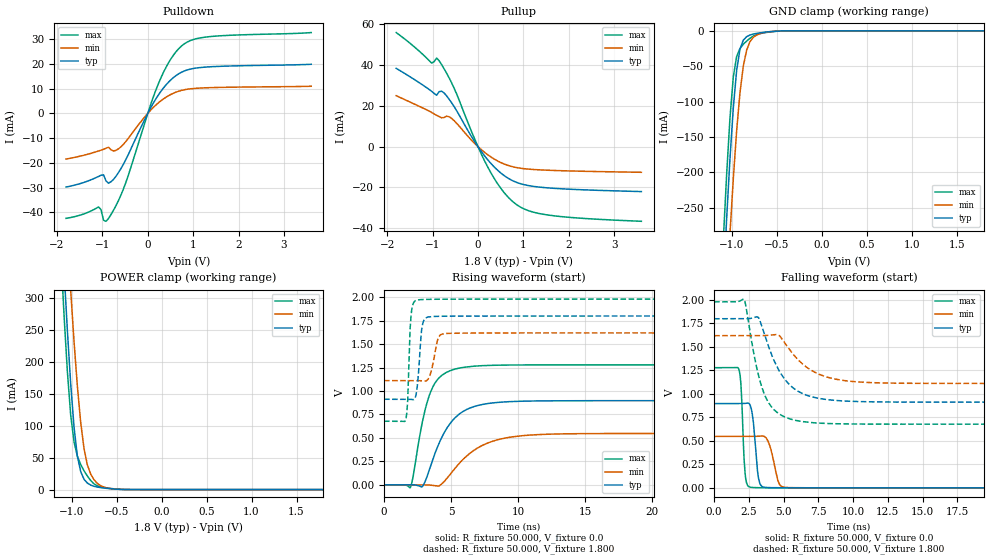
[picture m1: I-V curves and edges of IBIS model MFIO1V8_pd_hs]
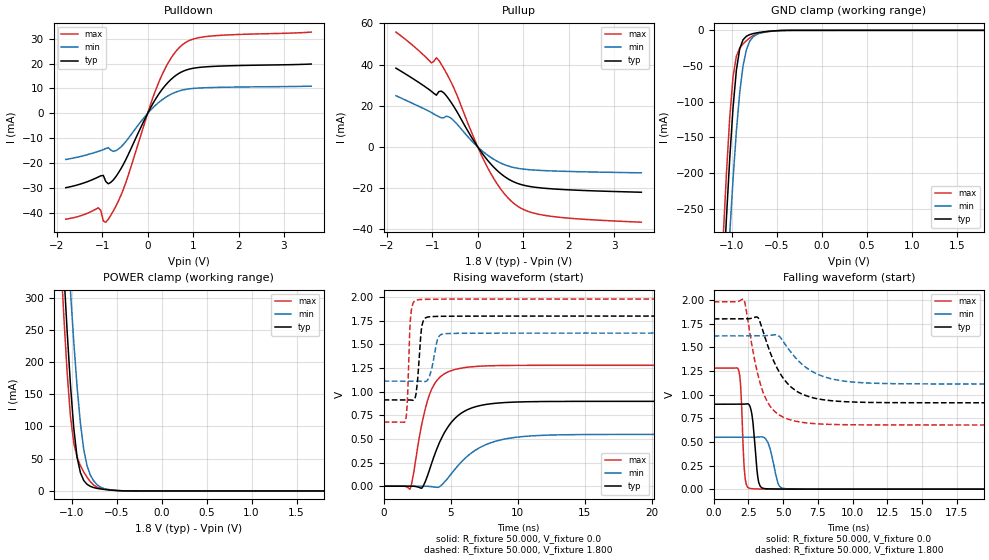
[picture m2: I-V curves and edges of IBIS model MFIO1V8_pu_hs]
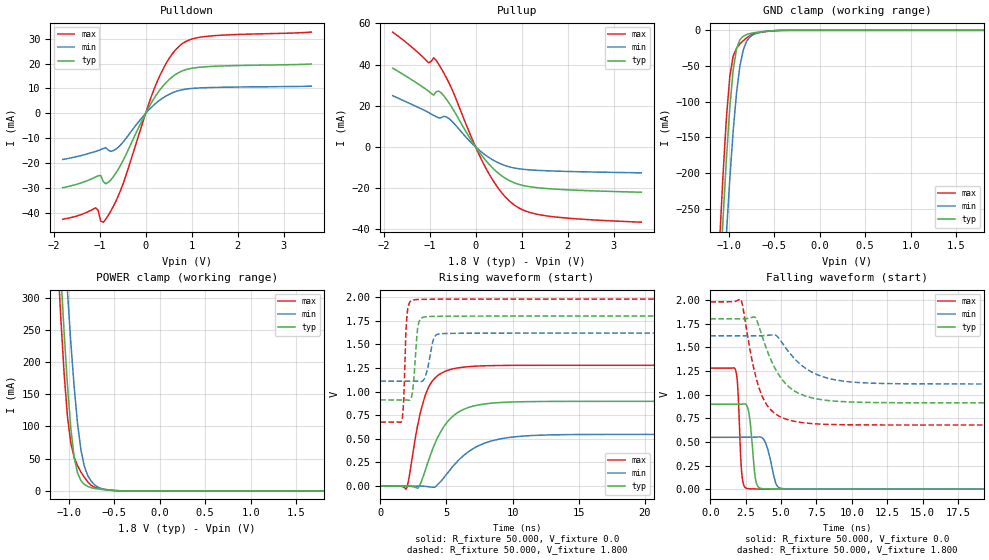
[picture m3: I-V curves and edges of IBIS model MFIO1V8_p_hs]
| IBIS file lpc55s6x_hlqfp100.ibs
[IBIS Ver]   5.0
[File name]   lpc55s6x_hlqfp100.ibs
[File Rev]   1.0
[Date]   January 29,2020
[Notes]   Rev History
|   1.0  initial release
[Disclaimer]   The model given below represents a 100-pin package.
[Copyright]   Copyright NXP 2020
|   Component lpc55s6x:hlqfp100
[Component] lpc55s6x
[Manufacturer] NXP
[Package]
|   typ   min   max
R_pkg   0.19438   0.14402   0.24011
L_pkg   4.719e-9   3.23e-9   5.804e-9
C_pkg   9.634e-13   4.793e-13   1.204e-12
[Pin]   Signal_name   model_name   R_pin   L_pin   C_pin
49   VBAT_DCDC   POWER   NA   NA   NA
50   VBAT_DCDC   POWER   NA   NA   NA
51   VBAT_PMU   POWER   NA   NA   NA
36   USB1_VBUS   POWER   NA   NA   NA
16   VDDA   POWER   NA   NA   NA
38   USB1_3V3   POWER   NA   NA   NA
96   USB0_3V3   POWER   NA   NA   NA
15   VDD   POWER   NA   NA   NA
25   VDD   POWER   NA   NA   NA
44   VDD   POWER   NA   NA   NA
63   VDD   POWER   NA   NA   NA
69   VDD   POWER   NA   NA   NA
75   VDD   POWER   NA   NA   NA
84   VDD   POWER   NA   NA   NA
95   VDD   POWER   NA   NA   NA
100   VDD   POWER   NA   NA   NA
39   VDD_PMU   POWER   NA   NA   NA
18   VREFN   NC   NA   NA   NA
17   VREFP   NC   NA   NA   NA
35   USB1_DM   NC   0.19961   3.9e-9   9.294e-13
34   USB1_DP   NC   0.20574   3.929e-9   9.444e-13
45   FB   NC   0.21411   3.71e-9   9.853e-13
48   LX   NC   0.14402   3.23e-9   1.143e-12
54   P0_0   gpio1v8   0.19671   5.046e-9   1.049e-12
7   P0_1   gpio1v8   0.18569   4.992e-9   9.758e-13
81   P0_2   gpio1v8   0.18955   4.93e-9   9.875e-13
83   P0_3   gpio1v8   0.20167   4.238e-9   9.373e-13
86   P0_4   gpio1v8   0.18453   4.604e-9   8.863e-13
88   P0_5   gpio1v8   0.17208   4.306e-9   4.861e-13
89   P0_6   gpio1v8   0.17688   4.76e-9   7.265e-13
6   P0_7   gpio1v8   0.18495   5.039e-9   9.877e-13
26   P0_8   gpio1v8   0.21082   5.764e-9   9.285e-13
55   P0_9   gpio1v8   0.18836   5.025e-9   1.013e-12
21   P0_10   gpio1v8   0.19767   4.742e-9   1.021e-12
13   P0_11   gpio1v8   0.16852   4.222e-9   4.793e-13
12   P0_12   gpio1v8   0.17445   4.737e-9   7.278e-13
71   P0_13   iicgpio1v8   0.20322   4.784e-9   1.026e-12
72   P0_14   iicgpio1v8   0.2062   5.002e-9   1.056e-12
22   P0_15   gpio1v8   0.20092   4.95e-9   1.063e-12
14   P0_16   gpio1v8   0.19182   3.934e-9   7.286e-13
8   P0_17   gpio1v8   0.18117   4.899e-9   9.571e-13
56   P0_18   gpio1v8   0.18284   4.955e-9   9.928e-13
90   P0_19   gpio1v8   0.17759   4.73e-9   8.974e-13
74   P0_20   gpio1v8   0.24011   4.357e-9   1.204e-12
76   P0_21   gpio1v8   0.21092   5.779e-9   9.242e-13
20   P0_22   gpio1v8   0.20457   4.183e-9   9.919e-13
78   P0_23   gpio1v8   0.19658   5.322e-9   1.084e-12
70   P0_24   gpio1v8   0.21211   4.242e-9   9.876e-13
79   P0_25   gpio1v8   0.19312   5.22e-9   1.048e-12
27   P0_26   gpio1v8   0.197   5.359e-9   1.171e-12
60   P0_27   gpio1v8   0.17389   4.719e-9   9.122e-13
66   P0_28   gpio1v8   0.18341   4.705e-9   9.109e-13
92   P0_9   gpio1v8   0.18226   4.694e-9   9.27e-13
23   P0_30   gpio1v8   0.21051   4.951e-9   1.105e-12
94   P0_31   gpio1v8   0.20907   4.051e-9   9.845e-13
11   P1_0   gpio1v8   0.17643   4.76e-9   9.003e-13
59   P1_1   gpio1v8   0.17508   4.772e-9   9.158e-13
61   P1_2   gpio1v8   0.17391   4.681e-9   9e-13
62   P1_3   gpio1v8   0.17584   4.65e-9   7.307e-13
1   P1_4   gpio1v8   0.21145   5.804e-9   9.228e-13
31   P1_5   gpio1v8   0.1979   4.791e-9   1.002e-12
5   P1_6   gpio1v8   0.19021   5.17e-9   1.023e-12
9   P1_7   gpio1v8   0.17814   4.834e-9   9.098e-13
10   P1_8   gpio1v8   0.1792   4.817e-9   9.052e-13
24   P1_9   gpio1v8   0.22787   4.483e-9   1.184e-12
40   P1_10   gpio1v8   0.19298   4.016e-9   8.906e-13
93   P1_11   gpio1v8   0.19014   4.583e-9   9.519e-13
67   P1_12   gpio1v8   0.19991   4.733e-9   9.253e-13
2   P1_13   gpio1v8   0.19954   5.432e-9   1.175e-12
57   P1_14   gpio1v8   0.17887   4.872e-9   9.721e-13
82   P1_15   gpio1v8   0.1908   4.68e-9   9.803e-13
43   P1_16   gpio1v8   0.20312   4.087e-9   9.402e-13
87   P1_17   gpio1v8   0.18016   4.71e-9   7.274e-13
64   P1_18   gpio1v8   0.17645   4.681e-9   7.229e-13
58   P1_19   gpio1v8   0.1767   4.814e-9   9.428e-13
4   P1_20   gpio1v8   0.19631   5.293e-9   1.056e-12
30   P1_21   gpio1v8   0.19856   5.07e-9   1.02e-12
41   P1_22   gpio1v8   0.18488   4.442e-9   9.08e-13
42   P1_23   gpio1v8   0.18716   4.441e-9   9.092e-13
3   P1_24   gpio1v8   0.20078   5.394e-9   1.079e-12
77   P1_25   gpio1v8   0.19946   5.414e-9   1.191e-12
68   P1_26   gpio1v8   0.20751   4.306e-9   9.447e-13
85   P1_27   gpio1v8   0.19867   4.289e-9   8.839e-13
73   P1_28   gpio1v8   0.21386   4.888e-9   1.092e-12
65   P1_29   gpio1v8   0.17885   4.696e-9   9.052e-13
80   P1_30   gpio1v8   0.18891   5.065e-9   1.012e-12
91   P1_31   gpio1v8   0.17881   4.709e-9   9.248e-13
32   RESETN   gpio1v8   0.2115   4.197e-9   9.778e-13
97   USB0_DP   NC   0.22563   4.185e-9   1.051e-12
98   USB0_DM   NC   0.23166   4.181e-9   1.087e-12
53   XTAL32K_N   NC   0.20814   4.918e-9   1.089e-12
52   XTAL32K_P   NC   0.23349   4.374e-9   1.189e-12
28   XTAL32M_N   NC   0.20639   5.416e-9   1.083e-12
29   XTAL32M_P   NC   0.20019   5.253e-9   1.052e-12
101   VSS   GND   NA   NA   NA
19   VSSA   GND   NA   NA   NA
33   USB1_VSS   GND   NA   NA   NA
37   USB1_VSS   GND   NA   NA   NA
47   VSS_DCDC   GND   NA   NA   NA
46   VSS_DCDC   GND   NA   NA   NA
99   USB0_VSS   GND   NA   NA   NA
|   Model Selector
[Model Selector] gpio1v8
MFIO1V8_pd_hs  EPUN=1 EPD=1 EHS=1
MFIO1V8_pd_ls  EPUN=1 EPD=1 EHS=0
MFIO1V8_pu_hs  EPUN=0 EPD=0 EHS=1
MFIO1V8_pu_ls  EPUN=0 EPD=0 EHS=0
MFIO1V8_p_hs  EPUN=1 EPD=0 EHS=1
MFIO1V8_p_ls  EPUN=1 EPD=0 EHS=0
MFIO1V8_r_hs  EPUN=0 EPD=1 EHS=1
MFIO1V8_r_ls  EPUN=0 EPD=1 EHS=0
[Model Selector] iicgpio1v8
IIC1V8_pd_hs  EGP=1 EPUN=1 EPD=1 EHS=1
IIC1V8_pd_ls  EGP=1 EPUN=1 EPD=1 EHS=0
IIC1V8_p_hs  EGP=1 EPUN=1 EPD=0 EHS=1
IIC1V8_p_ls  EGP=1 EPUN=1 EPD=0 EHS=0
IIC1V8_pu_hs  EGP=1 EPUN=0 EPD=0 EHS=1
IIC1V8_pu_ls  EGP=1 EPUN=0 EPD=0 EHS=0
IIC1V8_r_hs  EGP=1 EPUN=0 EPD=1 EHS=1
IIC1V8_r_ls  EGP=1 EPUN=0 EPD=1 EHS=0
IIC1V8_pd_iic_hs  EGP=0 ECS=0 EPUN=1 EPD=1
IIC1V8_p_iic_hs  EGP=0 ECS=0 EPUN=1 EPD=0
IIC1V8_pu_iic_hs  EGP=0 ECS=0 EPUN=0 EPD=0
IIC1V8_r_iic_hs  EGP=0 ECS=0 EPUN=0 EPD=1
IIC1V8_pd_iic_pu_hs  EGP=0 ECS=1 EPUN=1 EPD=1  SSEL=1
IIC1V8_p_iic_pu_hs  EGP=0 ECS=1 EPUN=1 EPD=0  SSEL=1
IIC1V8_pu_iic_pu_hs  EGP=0 ECS=1 EPUN=0 EPD=0  SSEL=1
IIC1V8_r_iic_pu_hs  EGP=0 ECS=1 EPUN=0 EPD=1  SSEL=1
| Models and submodels in the file (24): MFIO1V8_pd_hs (I/O), MFIO1V8_pd_ls (I/O), MFIO1V8_pu_hs (I/O), MFIO1V8_pu_ls (I/O), MFIO1V8_p_hs (I/O), MFIO1V8_p_ls (I/O), MFIO1V8_r_hs (I/O), MFIO1V8_r_ls (I/O), IIC1V8_pd_hs (I/O), IIC1V8_pd_ls (I/O), IIC1V8_p_hs (I/O), IIC1V8_p_ls (I/O), IIC1V8_pu_hs (I/O), IIC1V8_pu_ls (I/O), IIC1V8_r_hs (I/O), IIC1V8_r_ls (I/O), IIC1V8_pd_iic_hs (I/O_open_drain), IIC1V8_p_iic_hs (I/O_open_drain), IIC1V8_pu_iic_hs (I/O_open_drain), IIC1V8_r_iic_hs (I/O_open_drain), IIC1V8_pd_iic_pu_hs (I/O_open_drain), IIC1V8_p_iic_pu_hs (I/O_open_drain), IIC1V8_pu_iic_pu_hs (I/O_open_drain), IIC1V8_r_iic_pu_hs (I/O_open_drain)
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|   Model MFIO1V8_pd_hs
[Model] MFIO1V8_pd_hs
Model_type I/O
Polarity   Non-Inverting
Enable   Active-Low
Vinl =  0.540V
Vinh =  1.260V
Vmeas =  0.900V
Cref =  0.0F
Rref =  100.000
Vref =  0.0V
C_comp   2.019pF   1.989pF   2.068pF
C_comp_pullup   1.198pF   1.161pF   1.251pF
C_comp_pulldown   0.670pF   0.661pF   0.684pF
[Model Spec]
Vinh   1.260V   1.134V   1.386V
Vinl   0.540V   0.486V   0.594V
Vmeas   0.900V   0.810V   0.990V
Vref   0.0V   0.0V   0.0V
Cref   0.0F   0.0F   0.0F
Rref   100.000   100.000   100.000
[Temperature Range]   25.000   0.125k   -40.000
[Voltage Range]   1.800V   1.620V   1.980V
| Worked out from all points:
|   slope of the pulldown table from 0 to 0.27 V, typ, clamps not added: 32.2 ohm
|   slope of the pullup table from 0 to 0.27 V, typ, clamps not added: 34.3 ohm
|   GND clamp passes 1 mA (typ) near -0.56 V on its own axis
|   POWER clamp passes 1 mA (typ) near -0.54 V on its own axis
|   rising waveform, R_fixture 50.000, V_fixture 0.0: 20-80 % time 1.89ns typ, 2.69ns min, 1.21ns max; typ from 0 V to 0.897 V
|   rising waveform, R_fixture 50.000, V_fixture 1.800: 20-80 % time 276ps typ, 422ps min, 194ps max; typ from 0.912 V to 1.8 V
|   falling waveform, R_fixture 50.000, V_fixture 0.0: 20-80 % time 315ps typ, 502ps min, 217ps max; typ from 0.897 V to 0 V
|   falling waveform, R_fixture 50.000, V_fixture 1.800: 20-80 % time 1.84ns typ, 2.3ns min, 1.28ns max; typ from 1.8 V to 0.912 V
[Pulldown]
|Voltage   I(typ)   I(min)   I(max)
-1.8V     -29.75mA   -18.45mA   -42.39mA
-1.085V   -25.48mA   -15.2mA    -37.79mA
-1.03V    -24.99mA   -14.87mA   -38.88mA
-975mV    -24.83mA   -14.51mA   -43.15mA
-865mV    -28.18mA   -13.68mA   -42.43mA
-700mV    -25.38mA   -14.92mA   -37.23mA
-480mV    -18.54mA   -11.29mA   -27.73mA
235mV     7.474mA    4.265mA    12.03mA
510mV     13.55mA    7.648mA    22.01mA
785mV     16.96mA    9.446mA    27.8mA
1.39V     18.81mA    10.38mA    31.01mA
3.6V      19.8mA     10.93mA    32.61mA
[Pullup]
|Voltage   I(typ)   I(min)   I(max)
-1.8V     38.29mA    24.9mA     55.82mA
-1.02V    27.05mA    16.71mA    40.87mA
-910mV    25.14mA    15.31mA    43.32mA
-855mV    26.89mA    14.69mA    42.04mA
-745mV    26.24mA    14.22mA    38.06mA
-580mV    21.45mA    13.82mA    31.22mA
190mV     -5.761mA   -3.564mA   -8.914mA
520mV     -13.24mA   -7.997mA   -20.92mA
795mV     -17.02mA   -10.03mA   -27.47mA
1.07V     -18.92mA   -10.95mA   -31.04mA
1.51V     -20.18mA   -11.56mA   -33.41mA
3.6V      -22.04mA   -12.6mA    -36.6mA
[GND_clamp]
|Voltage   I(typ)   I(min)   I(max)
-1.8V     -2.463A    -2.494A    -2.446A
-1.097V   -357.7mA   -460.7mA   -294.8mA
-1.06V    -264.9mA   -370.9mA   -202.5mA
-1.023V   -180.4mA   -286.3mA   -122.9mA
-986mV    -108.7mA   -208.9mA   -65.05mA
-949mV    -56.06mA   -141.4mA   -36.24mA
-912mV    -25.87mA   -87.65mA   -25.01mA
-875mV    -13.21mA   -49.99mA   -19.06mA
-838mV    -8.315mA   -27.44mA   -14.52mA
-764mV    -4.558mA   -9.219mA   -7.395mA
-542mV    -813.9uA   -810.7uA   -1.086mA
1.8V      0A         0A         0A
[POWER_clamp]
|Voltage   I(typ)   I(min)   I(max)
-1.8V     2.577A     2.626A     2.553A
-1.123V   442.8mA    582.7mA    371.8mA
-1.086V   342mA      487.8mA    272.2mA
-1.049V   248.2mA    396.7mA    184.1mA
-1.012V   164.7mA    310.5mA    115.9mA
-975mV    97.4mA     231.2mA    74.47mA
-938mV    52.21mA    161.5mA    52.2mA
-864mV    16.15mA    64.06mA    29.43mA
-790mV    7.073mA    24.26mA    14.23mA
-679mV    3.152mA    6.087mA    4.407mA
-494mV    590.1uA    655.5uA    758.5uA
1.8V      0A         0A         0A
[Ramp]
| variable   typ   min   max
dV/dt_r   0.538/1.890n   0.328/2.680n   0.767/1.209n
dV/dt_f   0.532/1.835n   0.305/2.291n   0.781/1.275n
R_load = 50.000
[Rising Waveform]
R_fixture= 50.000
V_fixture= 0.0
V_fixture_min= 0.0
V_fixture_max= 0.0
|time   V(typ)   V(min)   V(max)
0s        6.721nV    117.6nV    4.416nV
1.96ns    159.2uV    -62.09nV   -31.69mV
2.85ns    -21.07mV   134.7uV    661mV
3.65ns    271.3mV    -6.708mV   1.047V
4.15ns    457.1mV    -8.65mV    1.146V
4.97ns    661.3mV    117.8mV    1.218V
6.65ns    830.9mV    361.7mV    1.264V
9.15ns    884.8mV    501.2mV    1.276V
13.74ns   896.1mV    543.8mV    1.278V
100ns     896.7mV    547.4mV    1.278V
[Rising Waveform]
R_fixture= 50.000
V_fixture= 1.800
V_fixture_min= 1.620
V_fixture_max= 1.980
|time   V(typ)   V(min)   V(max)
0s        911.9mV    1.111V     677.7mV
1.63ns    911.9mV    1.111V     697.7mV
1.77ns    912.1mV    1.111V     900.3mV
2.05ns    909.6mV    1.111V     1.849V
2.42ns    983.6mV    1.111V     1.967V
2.68ns    1.419V     1.11V      1.973V
3.06ns    1.772V     1.105V     1.976V
4.08ns    1.796V     1.575V     1.978V
4.84ns    1.798V     1.614V     1.979V
100ns     1.799V     1.619V     1.979V
[Falling Waveform]
R_fixture= 50.000
V_fixture= 0.0
V_fixture_min= 0.0
V_fixture_max= 0.0
|time   V(typ)   V(min)   V(max)
0s        896.7mV    547.4mV    1.278V
1.79ns    896.7mV    547.4mV    1.258V
1.93ns    896.6mV    547.4mV    1.106V
2.24ns    898.4mV    547.4mV    142.2mV
2.74ns    796.7mV    547.3mV    4.509mV
3.2ns     100.7mV    550.1mV    1.658mV
3.81ns    3.552mV    517mV      778.9uV
4.65ns    1.171mV    54.78mV    345.8uV
5.34ns    645.9uV    3.088mV    186.5uV
100ns     14.3nV     131.2nV    8.877nV
[Falling Waveform]
R_fixture= 50.000
V_fixture= 1.800
V_fixture_min= 1.620
V_fixture_max= 1.980
|time   V(typ)   V(min)   V(max)
0s        1.799V     1.619V     1.979V
2.17ns    1.799V     1.619V     2.003V
3.18ns    1.813V     1.619V     1.21V
3.88ns    1.522V     1.623V     915.7mV
4.62ns    1.262V     1.626V     793.3mV
5.16ns    1.14V      1.527V     750mV
6.98ns    971mV      1.252V     694.9mV
9.25ns    925.2mV    1.144V     680.9mV
13.25ns   913mV      1.113V     677.9mV
100ns     911.9mV    1.111V     677.7mV
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|   Model MFIO1V8_pu_hs
[Model] MFIO1V8_pu_hs
Model_type I/O
Polarity   Non-Inverting
Enable   Active-Low
Vinl =  0.540V
Vinh =  1.260V
Vmeas =  0.900V
Cref =  0.0F
Rref =  100.000
Vref =  0.0V
C_comp   2.019pF   1.989pF   2.068pF
C_comp_pullup   1.197pF   1.159pF   1.249pF
C_comp_pulldown   0.671pF   0.662pF   0.686pF
[Model Spec]
Vinh   1.260V   1.134V   1.386V
Vinl   0.540V   0.486V   0.594V
Vmeas   0.900V   0.810V   0.990V
Vref   0.0V   0.0V   0.0V
Cref   0.0F   0.0F   0.0F
Rref   100.000   100.000   100.000
[Temperature Range]   25.000   0.125k   -40.000
[Voltage Range]   1.800V   1.620V   1.980V
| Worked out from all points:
|   slope of the pulldown table from 0 to 0.27 V, typ, clamps not added: 32.2 ohm
|   slope of the pullup table from 0 to 0.27 V, typ, clamps not added: 34.3 ohm
|   GND clamp passes 1 mA (typ) near -0.56 V on its own axis
|   POWER clamp passes 1 mA (typ) near -0.54 V on its own axis
|   rising waveform, R_fixture 50.000, V_fixture 0.0: 20-80 % time 1.89ns typ, 2.68ns min, 1.21ns max; typ from 0.001 V to 0.898 V
|   rising waveform, R_fixture 50.000, V_fixture 1.800: 20-80 % time 275ps typ, 425ps min, 197ps max; typ from 0.913 V to 1.8 V
|   falling waveform, R_fixture 50.000, V_fixture 0.0: 20-80 % time 314ps typ, 505ps min, 216ps max; typ from 0.898 V to 0.001 V
|   falling waveform, R_fixture 50.000, V_fixture 1.800: 20-80 % time 1.84ns typ, 2.3ns min, 1.27ns max; typ from 1.8 V to 0.913 V
[Pulldown]
|Voltage   I(typ)   I(min)   I(max)
-1.8V     -29.75mA   -18.45mA   -42.39mA
-1.085V   -25.48mA   -15.2mA    -37.79mA
-1.03V    -24.99mA   -14.87mA   -38.88mA
-975mV    -24.83mA   -14.51mA   -43.15mA
-865mV    -28.18mA   -13.68mA   -42.43mA
-700mV    -25.38mA   -14.92mA   -37.23mA
-480mV    -18.54mA   -11.29mA   -27.73mA
235mV     7.474mA    4.265mA    12.03mA
510mV     13.55mA    7.648mA    22.01mA
785mV     16.96mA    9.446mA    27.8mA
1.39V     18.81mA    10.38mA    31.01mA
3.6V      19.8mA     10.93mA    32.61mA
[Pullup]
|Voltage   I(typ)   I(min)   I(max)
-1.8V     38.29mA    24.9mA     55.82mA
-1.02V    27.05mA    16.71mA    40.87mA
-910mV    25.14mA    15.31mA    43.32mA
-855mV    26.89mA    14.69mA    42.04mA
-745mV    26.24mA    14.22mA    38.06mA
-580mV    21.45mA    13.82mA    31.22mA
190mV     -5.761mA   -3.564mA   -8.914mA
520mV     -13.24mA   -7.997mA   -20.92mA
795mV     -17.02mA   -10.03mA   -27.47mA
1.07V     -18.92mA   -10.95mA   -31.04mA
1.51V     -20.18mA   -11.56mA   -33.41mA
3.6V      -22.04mA   -12.6mA    -36.6mA
[GND_clamp]
|Voltage   I(typ)   I(min)   I(max)
-1.8V     -2.463A    -2.494A    -2.446A
-1.097V   -357.7mA   -460.7mA   -294.9mA
-1.06V    -264.9mA   -371mA     -202.6mA
-1.023V   -180.4mA   -286.4mA   -122.9mA
-986mV    -108.7mA   -208.9mA   -65.09mA
-949mV    -56.09mA   -141.5mA   -36.28mA
-912mV    -25.91mA   -87.68mA   -25.06mA
-875mV    -13.24mA   -50.02mA   -19.11mA
-838mV    -8.35mA    -27.47mA   -14.57mA
-764mV    -4.593mA   -9.247mA   -7.441mA
-542mV    -849.5uA   -838.5uA   -1.132mA
1.8V      0A         0A         0A
[POWER_clamp]
|Voltage   I(typ)   I(min)   I(max)
-1.8V     2.577A     2.626A     2.553A
-1.123V   442.8mA    582.7mA    371.7mA
-1.086V   342mA      487.8mA    272.2mA
-1.049V   248.2mA    396.7mA    184.1mA
-1.012V   164.7mA    310.5mA    115.9mA
-975mV    97.36mA    231.1mA    74.42mA
-938mV    52.18mA    161.5mA    52.15mA
-864mV    16.11mA    64.03mA    29.39mA
-790mV    7.037mA    24.23mA    14.18mA
-679mV    3.116mA    6.059mA    4.361mA
-494mV    554.4uA    627.7uA    712.3uA
1.8V      0A         0A         0A
[Ramp]
| variable   typ   min   max
dV/dt_r   0.538/1.890n   0.329/2.680n   0.767/1.209n
dV/dt_f   0.532/1.835n   0.305/2.290n   0.781/1.276n
R_load = 50.000
[Rising Waveform]
R_fixture= 50.000
V_fixture= 0.0
V_fixture_min= 0.0
V_fixture_max= 0.0
|time   V(typ)   V(min)   V(max)
0s        630.6uV    679.1uV    587.5uV
1.96ns    789.2uV    678.8uV    -30.05mV
2.85ns    -19.7mV    812.3uV    661.1mV
3.62ns    261mV      -5.421mV   1.04V
4.13ns    453.5mV    -9.012mV   1.145V
4.91ns    652mV      107.5mV    1.216V
6.6ns     829.9mV    358mV      1.264V
9.06ns    885.4mV    500.2mV    1.277V
13.76ns   897.4mV    545.1mV    1.28V
100ns     898mV      548.7mV    1.28V
[Rising Waveform]
R_fixture= 50.000
V_fixture= 1.800
V_fixture_min= 1.620
V_fixture_max= 1.980
|time   V(typ)   V(min)   V(max)
0s        913.3mV    1.112V     678.9mV
1.63ns    913.3mV    1.112V     698.4mV
1.75ns    913.5mV    1.112V     853.9mV
2.02ns    911.7mV    1.112V     1.814V
2.4ns     967.4mV    1.112V     1.968V
2.67ns    1.397V     1.111V     1.974V
3.06ns    1.773V     1.107V     1.977V
4.07ns    1.797V     1.574V     1.979V
4.83ns    1.798V     1.615V     1.98V
100ns     1.8V       1.62V      1.98V
[Falling Waveform]
R_fixture= 50.000
V_fixture= 0.0
V_fixture_min= 0.0
V_fixture_max= 0.0
|time   V(typ)   V(min)   V(max)
0s        898mV      548.7mV    1.28V
1.79ns    898mV      548.7mV    1.259V
1.93ns    897.9mV    548.6mV    1.108V
2.24ns    899.8mV    548.7mV    143.9mV
2.76ns    775.9mV    548.5mV    5.275mV
3.23ns    78.56mV    551.7mV    2.369mV
3.84ns    4.35mV     511.3mV    1.439mV
4.67ns    1.941mV    48.66mV    967uV
5.32ns    1.374mV    4.206mV    798.7uV
100ns     630.7uV    679.1uV    587.5uV
[Falling Waveform]
R_fixture= 50.000
V_fixture= 1.800
V_fixture_min= 1.620
V_fixture_max= 1.980
|time   V(typ)   V(min)   V(max)
0s        1.8V       1.62V      1.98V
2.16ns    1.8V       1.62V      2.006V
3.18ns    1.814V     1.62V      1.212V
3.84ns    1.538V     1.623V     928.3mV
4.62ns    1.264V     1.627V     794.8mV
5.16ns    1.142V     1.528V     751.1mV
7.03ns    970.5mV    1.249V     695.5mV
9.17ns    927.3mV    1.147V     682.3mV
13.26ns   914.4mV    1.115V     679mV
100ns     913.3mV    1.112V     678.9mV
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|   Model MFIO1V8_p_hs
[Model] MFIO1V8_p_hs
Model_type I/O
Polarity   Non-Inverting
Enable   Active-Low
Vinl =  0.540V
Vinh =  1.260V
Vmeas =  0.900V
Cref =  0.0F
Rref =  100.000
Vref =  0.0V
C_comp   2.019pF   1.989pF   2.068pF
C_comp_pullup   1.197pF   1.160pF   1.250pF
C_comp_pulldown   0.671pF   0.662pF   0.686pF
[Model Spec]
Vinh   1.260V   1.134V   1.386V
Vinl   0.540V   0.486V   0.594V
Vmeas   0.900V   0.810V   0.990V
Vref   0.0V   0.0V   0.0V
Cref   0.0F   0.0F   0.0F
Rref   100.000   100.000   100.000
[Temperature Range]   25.000   0.125k   -40.000
[Voltage Range]   1.800V   1.620V   1.980V
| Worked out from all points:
|   slope of the pulldown table from 0 to 0.27 V, typ, clamps not added: 32.2 ohm
|   slope of the pullup table from 0 to 0.27 V, typ, clamps not added: 34.3 ohm
|   GND clamp passes 1 mA (typ) near -0.56 V on its own axis
|   POWER clamp passes 1 mA (typ) near -0.54 V on its own axis
|   rising waveform, R_fixture 50.000, V_fixture 0.0: 20-80 % time 1.89ns typ, 2.68ns min, 1.21ns max; typ from 0 V to 0.897 V
|   rising waveform, R_fixture 50.000, V_fixture 1.800: 20-80 % time 278ps typ, 422ps min, 192ps max; typ from 0.913 V to 1.8 V
|   falling waveform, R_fixture 50.000, V_fixture 0.0: 20-80 % time 314ps typ, 511ps min, 215ps max; typ from 0.897 V to 0 V
|   falling waveform, R_fixture 50.000, V_fixture 1.800: 20-80 % time 1.84ns typ, 2.3ns min, 1.28ns max; typ from 1.8 V to 0.913 V
[Pulldown]
|Voltage   I(typ)   I(min)   I(max)
-1.8V     -29.75mA   -18.45mA   -42.39mA
-1.085V   -25.48mA   -15.2mA    -37.79mA
-1.03V    -24.99mA   -14.87mA   -38.88mA
-975mV    -24.83mA   -14.51mA   -43.15mA
-865mV    -28.18mA   -13.68mA   -42.43mA
-700mV    -25.38mA   -14.92mA   -37.23mA
-480mV    -18.54mA   -11.29mA   -27.73mA
235mV     7.474mA    4.265mA    12.03mA
510mV     13.55mA    7.648mA    22.01mA
785mV     16.96mA    9.446mA    27.8mA
1.39V     18.81mA    10.38mA    31.01mA
3.6V      19.8mA     10.93mA    32.61mA
[Pullup]
|Voltage   I(typ)   I(min)   I(max)
-1.8V     38.29mA    24.9mA     55.82mA
-1.02V    27.05mA    16.71mA    40.87mA
-910mV    25.14mA    15.31mA    43.32mA
-855mV    26.89mA    14.69mA    42.04mA
-745mV    26.24mA    14.22mA    38.06mA
-580mV    21.45mA    13.82mA    31.22mA
190mV     -5.761mA   -3.564mA   -8.914mA
520mV     -13.24mA   -7.997mA   -20.92mA
795mV     -17.02mA   -10.03mA   -27.47mA
1.07V     -18.92mA   -10.95mA   -31.04mA
1.51V     -20.18mA   -11.56mA   -33.41mA
3.6V      -22.04mA   -12.6mA    -36.6mA
[GND_clamp]
|Voltage   I(typ)   I(min)   I(max)
-1.8V     -2.463A    -2.494A    -2.446A
-1.097V   -357.7mA   -460.7mA   -294.8mA
-1.06V    -264.9mA   -370.9mA   -202.5mA
-1.023V   -180.4mA   -286.3mA   -122.9mA
-986mV    -108.6mA   -208.9mA   -65.04mA
-949mV    -56.05mA   -141.4mA   -36.22mA
-912mV    -25.86mA   -87.64mA   -25mA
-875mV    -13.2mA    -49.98mA   -19.05mA
-838mV    -8.305mA   -27.43mA   -14.51mA
-764mV    -4.549mA   -9.211mA   -7.385mA
-542mV    -805.6uA   -803.8uA   -1.077mA
1.8V      0A         0A         0A
[POWER_clamp]
|Voltage   I(typ)   I(min)   I(max)
-1.8V     2.577A     2.626A     2.553A
-1.123V   442.8mA    582.7mA    371.7mA
-1.086V   342mA      487.8mA    272.1mA
-1.049V   248.2mA    396.6mA    184.1mA
-1.012V   164.7mA    310.5mA    115.9mA
-975mV    97.36mA    231.1mA    74.41mA
-938mV    52.17mA    161.5mA    52.14mA
-864mV    16.1mA     64.02mA    29.38mA
-790mV    7.028mA    24.22mA    14.17mA
-679mV    3.108mA    6.053mA    4.351mA
-494mV    546.6uA    621.4uA    702.9uA
1.8V      0A         0A         0A
[Ramp]
| variable   typ   min   max
dV/dt_r   0.538/1.892n   0.329/2.683n   0.768/1.210n
dV/dt_f   0.532/1.838n   0.305/2.294n   0.781/1.277n
R_load = 50.000
[Rising Waveform]
R_fixture= 50.000
V_fixture= 0.0
V_fixture_min= 0.0
V_fixture_max= 0.0
|time   V(typ)   V(min)   V(max)
0s        7.051nV    120nV      4.667nV
1.96ns    159.3uV    -60nV      -31.77mV
2.85ns    -21.07mV   134.7uV    659.8mV
3.66ns    277.4mV    -6.745mV   1.05V
4.15ns    457.5mV    -8.707mV   1.146V
5.02ns    670.7mV    126mV      1.221V
6.67ns    832.3mV    364.4mV    1.265V
9.24ns    886mV      503.8mV    1.277V
13.74ns   896.7mV    544.2mV    1.279V
100ns     897.3mV    547.8mV    1.279V
[Rising Waveform]
R_fixture= 50.000
V_fixture= 1.800
V_fixture_min= 1.620
V_fixture_max= 1.980
|time   V(typ)   V(min)   V(max)
0s        912.6mV    1.112V     678.1mV
1.63ns    912.6mV    1.112V     697.9mV
1.77ns    912.8mV    1.112V     903.5mV
2.03ns    910.9mV    1.112V     1.828V
2.4ns     967.2mV    1.112V     1.967V
2.66ns    1.375V     1.111V     1.974V
3ns       1.761V     1.107V     1.977V
4.06ns    1.797V     1.57V      1.979V
4.83ns    1.798V     1.615V     1.979V
100ns     1.8V       1.62V      1.98V
[Falling Waveform]
R_fixture= 50.000
V_fixture= 0.0
V_fixture_min= 0.0
V_fixture_max= 0.0
|time   V(typ)   V(min)   V(max)
0s        897.3mV    547.8mV    1.279V
1.79ns    897.3mV    547.8mV    1.258V
1.96ns    897.2mV    547.8mV    1.035V
2.25ns    899.3mV    547.8mV    128.7mV
2.75ns    785.4mV    547.7mV    4.896mV
3.23ns    77.6mV     550.8mV    1.878mV
3.83ns    3.769mV    511.9mV    959.3uV
4.67ns    1.371mV    47.13mV    456uV
5.37ns    779.8uV    3.194mV    261.7uV
100ns     14.63nV    133.6nV    9.13nV
[Falling Waveform]
R_fixture= 50.000
V_fixture= 1.800
V_fixture_min= 1.620
V_fixture_max= 1.980
|time   V(typ)   V(min)   V(max)
0s        1.8V       1.62V      1.98V
2.16ns    1.8V       1.62V      2.006V
3.19ns    1.813V     1.62V      1.204V
3.83ns    1.543V     1.623V     931.6mV
4.63ns    1.261V     1.626V     793.3mV
5.2ns     1.135V     1.52V      748.4mV
7.09ns    968mV      1.244V     694.1mV
9.25ns    926.1mV    1.145V     681.3mV
13.38ns   913.7mV    1.114V     678.3mV
100ns     912.6mV    1.112V     678.1mV
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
